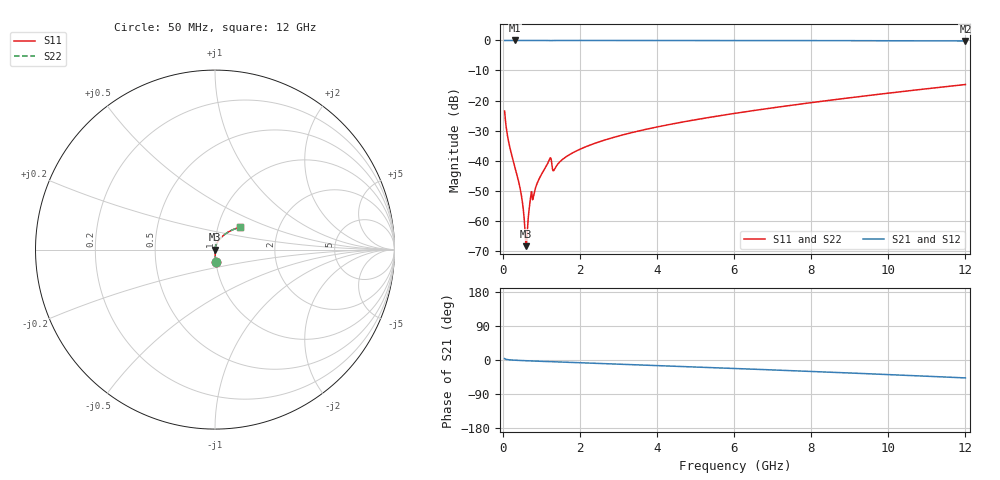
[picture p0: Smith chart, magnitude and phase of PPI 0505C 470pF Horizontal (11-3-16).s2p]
# MHz S MA R 50
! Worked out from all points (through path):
!   1601 points, 50 MHz to 12 GHz, reference 50 ohm
!   highest |S21| = 0.00 dB at 311.4 MHz (marker M1); lowest = -0.2 dB at 12 GHz (marker M2)
!   group delay of S21, straight-line fit = 10.9 ps
!   lowest |S11| = -68.5 dB at 610.2 MHz (marker M3), VSWR 1.00, Z = 50 + j0.000869 ohm
!   |S11| at or under -10 dB: start of sweep to end of sweep
!   |S22| runs from -68.5 to -14.7 dB; largest |S21 - S12| = 0
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50  0.06705 -86.2  0.9976 3.7  0.9976 3.7  0.06705 -86.2
169.5  0.01845 -88.7  0.9996 0.5  0.9996 0.5  0.01845 -88.7
311.4062  0.008091 -88.5  0.9997 -0.5  0.9997 -0.5  0.008091 -88.5
460.7812  0.003223 -85.4  0.9996 -1.3  0.9996 -1.3  0.003223 -85.4
513.0625  0.002001 -81.6  0.9996 -1.5  0.9996 -1.5  0.002001 -81.6
572.8125  0.000799 -64.8  0.9996 -1.8  0.9996 -1.8  0.000799 -64.8
610.1562  0.0003765 1.3  0.9996 -1.9  0.9996 -1.9  0.0003765 1.3
647.5  0.0008362 59.6  0.9996 -2.1  0.9996 -2.1  0.0008362 59.6
699.7812  0.001846 72.5  0.9995 -2.3  0.9995 -2.3  0.001846 72.5
752.0625  0.003028 55.4  0.9983 -2.5  0.9983 -2.5  0.003028 55.4
938.7812  0.00487 81.2  0.9995 -3.3  0.9995 -3.3  0.00487 81.2
1192.719  0.009733 76.4  0.9983 -4.3  0.9983 -4.3  0.009733 76.4
1230.062  0.011 67.4  0.9965 -4.5  0.9965 -4.5  0.011 67.4
1349.562  0.007271 73.2  0.9984 -4.7  0.9984 -4.7  0.007271 73.2
1596.031  0.011 81.0  0.9992 -5.7  0.9992 -5.7  0.011 81.0
2044.156  0.01587 80.5  0.9991 -7.4  0.9991 -7.4  0.01587 80.5
2880.656  0.02438 78.0  0.9989 -10.5  0.9989 -10.5  0.02438 78.0
4038.312  0.03668 74.0  0.9983 -14.8  0.9983 -14.8  0.03668 74.0
6025  0.06122 66.8  0.9969 -22.4  0.9969 -22.4  0.06122 66.8
8019.156  0.0925 59.1  0.9942 -30.3  0.9942 -30.3  0.0925 59.1
10013.31  0.1329 51.0  0.9893 -38.5  0.9893 -38.5  0.1329 51.0
12000  0.1847 42.3  0.9806 -47.3  0.9806 -47.3  0.1847 42.3
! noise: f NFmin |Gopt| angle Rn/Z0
50  0.0002978  0.8265  0.2287  0.0003609
1372  0.004126  0.6834  4.313  0.002523
2701  0.004383  0.484  8.183  0.001445
4031  0.00583  0.4404  11.96  0.001712
5360  0.007212  0.4131  15.58  0.001969
6682  0.008561  0.3956  19.01  0.002225
8012  0.009923  0.385  22.3  0.002496
9341  0.01132  0.3801  25.43  0.002789
1.067e+04  0.01278  0.38  28.41  0.003117
1.2e+04  0.01432  0.3844  31.28  0.003492
